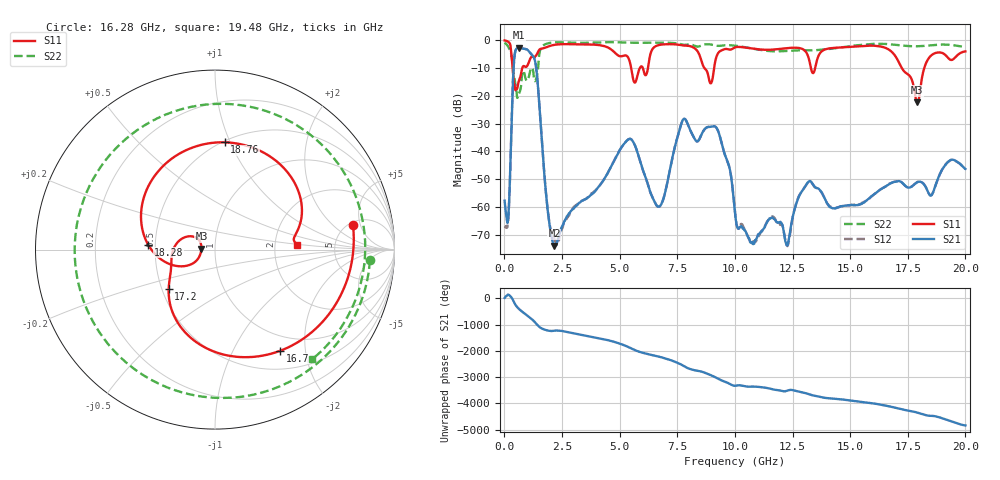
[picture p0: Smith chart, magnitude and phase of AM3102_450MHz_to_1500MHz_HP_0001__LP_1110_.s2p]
!Agilent Technologies,E8364B,MY43040894,A.07.50.67
!Agilent E8364B: A.07.50.67
!Date: Thursday, January 11, 2018 05:22:58
!Correction: S11(Full 2 Port(1,2))
!S21(Full 2 Port(1,2))
!S12(Full 2 Port(1,2))
!S22(Full 2 Port(1,2))
!S2P File: Measurements: S11, S21, S12, S22:
# Hz S  dB  R 50
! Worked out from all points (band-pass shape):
!   1601 points, 10 MHz to 20 GHz, reference 50 ohm
!   highest |S21| = -2.63 dB at 634.7 MHz (marker M1); lowest = -74.0 dB at 2.171 GHz (marker M2)
!   |S21| within 3 dB of the highest: 440.8 MHz to 1.234 GHz (792.8 MHz wide, 94.7 % of centre)
!   lowest |S11| = -22.4 dB at 17.91 GHz (marker M3), VSWR 1.16, Z = 43 + j0.467 ohm
!   |S11| at or under -10 dB: 357.3 MHz to 775.9 MHz (418.6 MHz wide, 73.9 % of centre); 8.678 GHz to 9.098 GHz (420.8 MHz wide, 4.73 % of centre); 17.24 GHz to 18.21 GHz (971.2 MHz wide, 5.48 % of centre)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
!   |S22| runs from -20.7 to -0.7 dB; largest |S21 - S12| = 0.0041
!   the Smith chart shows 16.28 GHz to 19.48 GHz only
!   S11 on the Smith chart (normalised r, x): 16.28 GHz: 5.43, +3.78; 16.7 GHz: 0.76, -1.56; 17.2 GHz: 0.54, -0.27; 18.28 GHz: 0.46, +0.03; 18.76 GHz: 0.51, +0.95; 19.48 GHz: 2.67, +0.18
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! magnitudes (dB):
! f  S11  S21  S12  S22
! 10 MHz  0.0  -57.8  -67.0  -0.9
! 434.8 MHz  -16.1  -6.1  -6.1  -13.6
! 634.7 MHz  -14.6  -2.6  -2.6  -19.2
! 1.334 GHz  -5.9  -7.6  -7.6  -14.7
! 2.171 GHz  -1.6  -74.0  -71.9  -0.8
! 3.346 GHz  -1.5  -57.9  -57.9  -0.9
! 5.445 GHz  -7.9  -35.5  -35.5  -0.8
! 6.682 GHz  -1.7  -60.0  -60.0  -0.8
! 7.806 GHz  -1.9  -28.3  -28.3  -1.6
! 9.23 GHz  -5.3  -31.9  -31.9  -2.0
! 10.01 GHz  -2.6  -62.2  -61.8  -1.9
! 12.27 GHz  -2.8  -73.9  -74.0  -3.8
! 13.34 GHz  -11.3  -51.3  -51.4  -3.6
! 16.28 GHz  -2.2  -54.0  -54.0  -1.3
! 16.68 GHz  -3.3  -51.9  -51.8  -1.4
! 16.7 GHz  -3.5  -51.8  -51.7  -1.4
! 17.2 GHz  -9.4  -51.0  -51.0  -1.8
! 17.91 GHz  -22.4  -51.2  -51.0  -2.1
! 18.28 GHz  -8.5  -52.8  -52.8  -2.0
! 18.76 GHz  -4.4  -50.9  -50.9  -1.6
! 19.48 GHz  -6.8  -43.1  -43.1  -1.8
! 20 GHz  -4.0  -46.3  -46.4  -2.4
